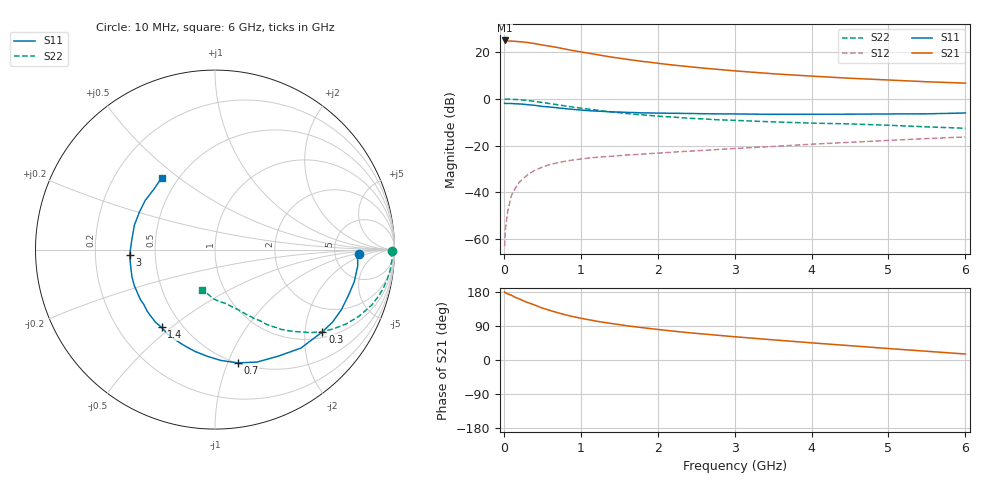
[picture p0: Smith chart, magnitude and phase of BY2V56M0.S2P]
! SIEMENS Small Signal Semiconductors
! BFY420
! Si NPN RF SIEGET Grounded Emitter Transistor in MICRO-X
! VCE = 2.5 V  IC = 6 mA
! Common Emitter S-Parameters:  October  1996
# GHz  S  MA  R  50
!  f  S11  S21  S12  S22
! GHz  MAG  ANG  MAG  ANG  MAG  ANG  MAG  ANG
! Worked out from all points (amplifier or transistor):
!   36 points, 10 MHz to 6 GHz, reference 50 ohm
!   highest |S21| = 25.0 dB at 10 MHz (marker M1)
!   |S21| within 3 dB of that: start of sweep to 692.3 MHz
!   unconditionally stable (mu >= 1): 3.011 GHz to end of sweep
!   at 250 MHz: K = 0.13, MSG = 29.3 dB, |S12| = -34.2 dB
!   at 1.4 GHz: K = 0.59, MSG = 21.2 dB, |S12| = -24.6 dB
!   at 6 GHz: K = 1.12, MAG = 9.4 dB, |S12| = -16.3 dB
!   S11 on the Smith chart (normalised r, x): 10 MHz: 9.03, -1.22; 300 MHz: 1.16, -2.47; 700 MHz: 0.50, -1.09; 1.4 GHz: 0.39, -0.46; 3 GHz: 0.35, -0.03; 6 GHz: 0.41, +0.43
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0.01  0.8038 -1.7  17.86 179.6  0.0007 85.1  0.9887 -0.6
0.02  0.7953 -2.7  17.72 177.4  0.0016 77.5  0.9825 -1.3
0.05  0.8004 -6.5  17.39 174.5  0.0039 87.0  0.9875 -3.3
0.1  0.7961 -13.0  17.29 170.8  0.0087 82.8  0.9829 -6.7
0.15  0.7858 -19.2  17.08 165.2  0.0122 79.5  0.9727 -10.1
0.2  0.7797 -25.5  16.82 161.4  0.0163 78.1  0.9609 -13.2
0.25  0.7696 -31.6  16.55 156.6  0.0194 73.0  0.9442 -16.4
0.3  0.7539 -37.4  16.18 152.4  0.0231 71.0  0.9271 -19.4
0.4  0.7282 -48.9  15.31 145.1  0.0294 66.1  0.8834 -24.9
0.5  0.69 -59.4  14.26 137.0  0.0346 61.5  0.8383 -29.7
0.6  0.6689 -69.5  13.46 130.8  0.0393 57.8  0.7926 -33.9
0.7  0.6438 -78.6  12.58 124.8  0.043 54.2  0.7484 -37.7
0.9  0.5958 -94.2  10.83 114.5  0.0492 48.9  0.6675 -43.5
1.1  0.5603 -108.2  9.542 106.4  0.0539 46.0  0.6037 -48.4
1.4  0.5257 -124.5  7.853 96.3  0.059 42.9  0.5292 -53.7
1.7  0.5099 -138.0  6.7 87.9  0.064 41.4  0.4674 -57.8
2.2  0.4923 -156.0  5.302 76.2  0.0723 39.4  0.4077 -63.6
3  0.4764 -176.4  3.987 61.4  0.0864 38.0  0.3471 -70.9
3.5  0.4665 172.7  3.455 53.2  0.0958 36.6  0.3217 -75.4
4.5  0.4703 153.5  2.767 37.8  0.1175 32.2  0.2909 -85.1
5.5  0.479 135.1  2.327 23.0  0.1413 26.2  0.2515 -98.9
6  0.4988 126.6  2.176 15.8  0.1529 22.5  0.2347 -107.6
